(* Logix 5000 AddOnInstructionDefinition export EH_Dosimass_IOL; software revision 38.00 *)

TYPE EH_CommAOI_Data :
STRUCT
   Device_Comm_Error : BOOL;
   CommSuccess : BOOL;
   CommFailed : BOOL;
   CommTimeOut : BOOL;
   StateDone : BOOL;
   NewState : BOOL;
   OldState : SINT;
   PortSize : SINT;
   DevicePort : SINT;
   MaxState : SINT;
   State : SINT;
   VendorID : INT;
   DeviceID : DINT;
   CyclicData : INT[16];
   AcyclicData : DINT[8];
   ReplayIndex : INT;
   AOI_Diagnostic : DINT;
   ConnectionStatus : DINT;
   OutputData : INT[16];
END_STRUCT
END_TYPE

ADD_ON_INSTRUCTION EH_Dosimass_IOL   (* revision 1.1, vendor Endress+Hauser *)
// Dosimass D8AB Rev 1 IO-Link
// Revision note:
// 1.1 Changed the Datatype from Unsigned to Signed
// ZeroPoint adjustment update
// Add Disconnect check
// Add condition PulseSimulation
VAR_IN_OUT
   DataToSend : INT[10]; {required}
   CommAOIBusy : DINT; {required}
   ActiveComPort : DINT; {required}
   DeviceAOISendRequest : DINT; {required}
   CommError : INT; {required}
   DeviceData : EH_CommAOI_Data; {required}
END_VAR
VAR_INPUT
   iSetPulseSimulation : BOOL; {visible}
   iSimulationOnOff : BOOL; {visible}
   iAmountPulses : INT; {visible}
   iSetTotalizerPresetValue : BOOL; {visible}
   iTotalizer1PresetValue : REAL; {visible}
   iTotalizer_Hold : BOOL; {visible}
   iTotalizer_ResetTotalize : BOOL; {visible}
   iTotalizer_ResetHold : BOOL; {visible}
   iTotalizer_Totalize : BOOL; {visible}
   iParameterize : BOOL; {visible}
   iFlowDamping : REAL; {visible}
   iPressureShockSupression : REAL; {visible}
   iLowFlowCutoffValue : REAL; {visible}
   iFlowOverride : BOOL; {visible}
   iStartZeroPointAdjustment : BOOL; {visible}
END_VAR
VAR_OUTPUT
   qVendor_ID : DINT; {access Read Only, visible}
   qDevice_ID : DINT; {access Read Only, visible}
   qMassFlow : REAL; {visible}
   qDensity : REAL; {visible}
   qTemperature : REAL; {visible}
   qTotalizer1 : REAL; {access Read Only, visible}
   qExtendedDeviceStatus : INT; {access Read Only, visible}
   qZeroPointStatus : SINT; {access Read Only, visible}
   qReadProgress : SINT; {access Read Only, visible}
   qSSC1_1 : BOOL; {access Read Only, visible}
   qSSC1_2 : BOOL; {access Read Only, visible}
   qSSC2_1 : BOOL; {access Read Only, visible}
   qSSC2_2 : BOOL; {access Read Only, visible}
   qSSC3_1 : BOOL; {access Read Only, visible}
   qSSC3_2 : BOOL; {access Read Only, visible}
   qSSC4_1 : BOOL; {access Read Only, visible}
   qSSC4_2 : BOOL; {access Read Only, visible}
   qAOI_Diagnostic : DINT; {access Read Only, visible}
END_VAR
VAR_IN_OUT
   qAOI_Diagnostic_String : STRING; {required}
END_VAR
VAR_OUTPUT
   qActual_Diagnostics_Code : DINT; {access Read Only, visible}
END_VAR
VAR_IN_OUT
   qActual_Diagnostics_String : STRING; {required}
END_VAR
VAR_OUTPUT
   qLast_Diagnostics_Code : DINT; {visible}
END_VAR
VAR_IN_OUT
   qLast_Diagnostics_String : STRING; {required}
END_VAR
VAR_OUTPUT
   qCommError : DINT; {access None}
   qCommunicationBusy : DINT; {access Read Only, visible}
   qDeviceConnectionError : BOOL; {access Read Only, visible}
END_VAR
VAR
   Temp_DINT : DINT; {access None}
   CMD_Index : INT; {access None}
   CMD_Subindex : INT; {access None}
   CMD_ByteLength : INT; {access None}
   oldCondStatus : INT; {access None}
   SetSimulation : SINT; {access None}
   SetTotalizer : SINT; {access None}
   oldSetTotalizer : SINT; {access None}
   oldStartZeroPointAdjustment : SINT; {access None}
   Trigger : BOOL; {access None}
   CMD_Rd : BOOL; {access None}
   CMD_Wr : BOOL; {access None}
   SimulationDINT : DINT; {access None}
   AOI_Prio : BOOL; {access None}
   StateMin : DINT; {access None}
   firstTimeDone : BOOL; {access None}
   CondStatusChanged : BOOL; {access None}
   Calc_MassFlow : DINT; {access None}
   Calc_Density : DINT; {access None}
   Calc_Temperature : DINT; {access None}
   Calc_Totalizer1 : DINT; {access None}
   Calc_ExtendedDeviceStatus : DINT; {access None}
   CondStatusActive : BOOL; {access None}
   ActiveAOI : BOOL; {access None}
   TotActive : BOOL; {access None}
   Skip : BOOL; {access None}
   StartZeroPointAdjustment : SINT; {access None}
   Parameterize : SINT; {access None}
   oldParameterize : SINT; {access None}
   oldSetPulseSimulation : SINT; {access None}
   TotChanged : BOOL; {access None}
   DeviceID : DINT; {access None}
   SetPulseSimulation : SINT; {access None}
   zeroPointStatus : SINT; {access None}
   StartZeroPointAdjustmentChanged : BOOL; {access None}
   ParameterizeChanged : BOOL; {access None}
   PulseSimChanged : BOOL; {access None}
   TRUE : BOOL := 1; {access None}
   FALSE : BOOL; {access None}
   ParameterizeActive : BOOL; {access None}
   PulseSimActive : BOOL; {access None}
   ZeroPointActive : BOOL; {access None}
   StandardTimer : FBD_TIMER; {access None}
   temp_string1 : STRING; {access None}
   temp_string2 : STRING; {access None}
   onlyonce : BOOL; {access None}
END_VAR

ROUTINE Logic   (* structured text *)
// Picomag Communication via AL1323
   // =======================================================================
   // Endress+Hauser Digital Solutions
   // ©Copyright (2024) All Rights Reserved
   // =======================================================================
   // Name:                EH_Dosimass_IOL
   // Version:             1.1
   // Datum:               02.2026
   // Library:             01.01.00
   // Engineering:         Studio5000 V38.00.00
   // Author:              EH
   // =======================================================================
   
   qAOI_Diagnostic := DeviceData.AOI_Diagnostic;
   qCommunicationBusy := CommAOIBusy;
   DeviceID := 9729025;
   StateMin := 0;
   DeviceData.MaxState := 98;
   
   if DeviceData.DevicePort = 0 or DeviceData.DeviceID <> DeviceID or DeviceData.ConnectionStatus <> 1 then
   
   	qVendor_ID := DeviceData.VendorID;
   	qDevice_ID := DeviceData.DeviceID;
   	qMassFlow := 0;
   	qDensity := 0;
   	qTemperature := 0;
   	qTotalizer1	:= 0;
   	qExtendedDeviceStatus := 0;
   	qSSC1_1	:= FALSE;
   	qSSC1_2	:= FALSE;
   	qSSC2_1	:= FALSE;
   	qSSC2_2	:= FALSE;
   	qSSC3_1	:= FALSE;
   	qSSC3_2	:= FALSE;
   	qSSC4_1	:= FALSE;
   	qSSC4_2	:= FALSE;
   	qActual_Diagnostics_Code := 0;
   	qActual_Diagnostics_String := '';
   	qLast_Diagnostics_Code := 0;
   	qLast_Diagnostics_String := '';
   	qReadProgress := 0;
   	qZeroPointStatus := 0;
   	oldCondStatus := 0;
   	CondStatusChanged := FALSE;
   
   	if DeviceData.DevicePort = 0 then
   
   		qAOI_Diagnostic_String	:= 'Device Port is Zero';
   		DeviceData.AOI_Diagnostic.1 := TRUE;
   
   	elsif DeviceData.ConnectionStatus <> 1 then
   
   		qAOI_Diagnostic_String	:= 'No Device connected';
   		qDeviceConnectionError := TRUE;
   
   	elsif DeviceData.DeviceID <> DeviceID then
   
   		qAOI_Diagnostic_String	:= 'Wrong DeviceID';
   		DeviceData.AOI_Diagnostic.2 := TRUE;
   	end_if;
   
   else
   
   	if qActual_Diagnostics_Code = 0  then
   
   		qActual_Diagnostics_String	:= '--------';
   
   	end_if;
   
   	if qLast_Diagnostics_Code = 0 then
   
   		qLast_Diagnostics_String	:= '--------';
   
   	end_if;
   
   	qAOI_Diagnostic_String := '';
   	DeviceData.AOI_Diagnostic.1 := FALSE;
   	qDeviceConnectionError := FALSE;
   	DeviceData.AOI_Diagnostic.2  := FALSE;
   
   end_if;
   
   // Case device disconnected during communication to avoid blocking the communication
   if (DeviceData.AOI_Diagnostic.0 or qDeviceConnectionError or DeviceData.AOI_Diagnostic.2) and ActiveAOI and ActiveComPort = DeviceData.DevicePort and CommAOIBusy = 1 then
   
   	DeviceData.State := 0;
   	CommAOIBusy := 0;
   	DeviceAOISendRequest.[DeviceData.DevicePort] := 0;
   	ActiveComPort := 0;
   	ActiveAOI := 0;
   	DataToSend[0] := 0;
   	DataToSend[1] := 0;
   	DataToSend[2] := 0;
   	DataToSend[3] := 0;
   	DataToSend[4] := 0;
   	DataToSend[5] := 0;
   	DataToSend[6] := 0;
   	DataToSend[7] := 0;
   	DataToSend[8] := 0;
   	DataToSend[9] := 0;
   	DeviceData.StateDone := FALSE;
   	DeviceData.NewState := FALSE;
   	DeviceData.OldState := 0;
   	ActiveAOI := FALSE;
   
   end_if;
   
   if not DeviceData.AOI_Diagnostic.0
   	and not qDeviceConnectionError
   	and not DeviceData.AOI_Diagnostic.2
   	and DeviceData.DevicePort > 0 then
   
   	//*********************************
   	//Vendor ID
   	//*********************************
   
   		qVendor_ID := DeviceData.VendorID;
   
   	//*********************************
   	//Device ID
   	//*********************************
   
   		qDevice_ID := DeviceData.DeviceID;
   
   	//*********************************
   	// Dosimass
   	//*********************************
   
   		Calc_MassFlow				:= 0;
   		Calc_Density				:= 2;
   		Calc_Temperature			:= 4;
   		Calc_Totalizer1				:= 6;
   		Calc_ExtendedDeviceStatus	:= 8;
   
   	//*********************************
   	//Process MassFlow
   	//*********************************
   
   		Temp_DINT	 := DeviceData.CyclicData[Calc_MassFlow+1];
   		Temp_DINT.8	 := DeviceData.CyclicData[Calc_MassFlow+1].8;
   		Temp_DINT.9  := DeviceData.CyclicData[Calc_MassFlow+1].9;
   		Temp_DINT.10 := DeviceData.CyclicData[Calc_MassFlow+1].10;
   		Temp_DINT.11 := DeviceData.CyclicData[Calc_MassFlow+1].11;
   		Temp_DINT.12 := DeviceData.CyclicData[Calc_MassFlow+1].12;
   		Temp_DINT.13 := DeviceData.CyclicData[Calc_MassFlow+1].13;
   		Temp_DINT.14 := DeviceData.CyclicData[Calc_MassFlow+1].14;
   		Temp_DINT.15 := DeviceData.CyclicData[Calc_MassFlow+1].15;
   		Temp_DINT.16 := DeviceData.CyclicData[Calc_MassFlow].0;
   		Temp_DINT.17 := DeviceData.CyclicData[Calc_MassFlow].1;
   		Temp_DINT.18 := DeviceData.CyclicData[Calc_MassFlow].2;
   		Temp_DINT.19 := DeviceData.CyclicData[Calc_MassFlow].3;
   		Temp_DINT.20 := DeviceData.CyclicData[Calc_MassFlow].4;
   		Temp_DINT.21 := DeviceData.CyclicData[Calc_MassFlow].5;
   		Temp_DINT.22 := DeviceData.CyclicData[Calc_MassFlow].6;
   		Temp_DINT.23 := DeviceData.CyclicData[Calc_MassFlow].7;
   		Temp_DINT.24 := DeviceData.CyclicData[Calc_MassFlow].8;
   		Temp_DINT.25 := DeviceData.CyclicData[Calc_MassFlow].9;
   		Temp_DINT.26 := DeviceData.CyclicData[Calc_MassFlow].10;
   		Temp_DINT.27 := DeviceData.CyclicData[Calc_MassFlow].11;
   		Temp_DINT.28 := DeviceData.CyclicData[Calc_MassFlow].12;
   		Temp_DINT.29 := DeviceData.CyclicData[Calc_MassFlow].13;
   		Temp_DINT.30 := DeviceData.CyclicData[Calc_MassFlow].14;
   		Temp_DINT.31 := DeviceData.CyclicData[Calc_MassFlow].15;
   
   		COP(Temp_DINT,qMassFlow,1);
   
   	//*********************************
   	//Process Data Density
   	//*********************************
   
   		Temp_DINT	 := DeviceData.CyclicData[Calc_Density+1];
   		Temp_DINT.8	 := DeviceData.CyclicData[Calc_Density+1].8;
   		Temp_DINT.9	 := DeviceData.CyclicData[Calc_Density+1].9;
   		Temp_DINT.10 := DeviceData.CyclicData[Calc_Density+1].10;
   		Temp_DINT.11 := DeviceData.CyclicData[Calc_Density+1].11;
   		Temp_DINT.12 := DeviceData.CyclicData[Calc_Density+1].12;
   		Temp_DINT.13 := DeviceData.CyclicData[Calc_Density+1].13;
   		Temp_DINT.14 := DeviceData.CyclicData[Calc_Density+1].14;
   		Temp_DINT.15 := DeviceData.CyclicData[Calc_Density+1].15;
   		Temp_DINT.16 := DeviceData.CyclicData[Calc_Density].0;
   		Temp_DINT.17 := DeviceData.CyclicData[Calc_Density].1;
   		Temp_DINT.18 := DeviceData.CyclicData[Calc_Density].2;
   		Temp_DINT.19 := DeviceData.CyclicData[Calc_Density].3;
   		Temp_DINT.20 := DeviceData.CyclicData[Calc_Density].4;
   		Temp_DINT.21 := DeviceData.CyclicData[Calc_Density].5;
   		Temp_DINT.22 := DeviceData.CyclicData[Calc_Density].6;
   		Temp_DINT.23 := DeviceData.CyclicData[Calc_Density].7;
   		Temp_DINT.24 := DeviceData.CyclicData[Calc_Density].8;
   		Temp_DINT.25 := DeviceData.CyclicData[Calc_Density].9;
   		Temp_DINT.26 := DeviceData.CyclicData[Calc_Density].10;
   		Temp_DINT.27 := DeviceData.CyclicData[Calc_Density].11;
   		Temp_DINT.28 := DeviceData.CyclicData[Calc_Density].12;
   		Temp_DINT.29 := DeviceData.CyclicData[Calc_Density].13;
   		Temp_DINT.30 := DeviceData.CyclicData[Calc_Density].14;
   		Temp_DINT.31 := DeviceData.CyclicData[Calc_Density].15;
   
   		COP(Temp_DINT,qDensity,1);
   
   	//*********************************
   	//Process Data Temperature
   	//*********************************
   
   		Temp_DINT	 := DeviceData.CyclicData[Calc_Temperature+1];
   		Temp_DINT.8	 := DeviceData.CyclicData[Calc_Temperature+1].8;
   		Temp_DINT.9	 := DeviceData.CyclicData[Calc_Temperature+1].9;
   		Temp_DINT.10 := DeviceData.CyclicData[Calc_Temperature+1].10;
   		Temp_DINT.11 := DeviceData.CyclicData[Calc_Temperature+1].11;
   		Temp_DINT.12 := DeviceData.CyclicData[Calc_Temperature+1].12;
   		Temp_DINT.13 := DeviceData.CyclicData[Calc_Temperature+1].13;
   		Temp_DINT.14 := DeviceData.CyclicData[Calc_Temperature+1].14;
   		Temp_DINT.15 := DeviceData.CyclicData[Calc_Temperature+1].15;
   		Temp_DINT.16 := DeviceData.CyclicData[Calc_Temperature].0;
   		Temp_DINT.17 := DeviceData.CyclicData[Calc_Temperature].1;
   		Temp_DINT.18 := DeviceData.CyclicData[Calc_Temperature].2;
   		Temp_DINT.19 := DeviceData.CyclicData[Calc_Temperature].3;
   		Temp_DINT.20 := DeviceData.CyclicData[Calc_Temperature].4;
   		Temp_DINT.21 := DeviceData.CyclicData[Calc_Temperature].5;
   		Temp_DINT.22 := DeviceData.CyclicData[Calc_Temperature].6;
   		Temp_DINT.23 := DeviceData.CyclicData[Calc_Temperature].7;
   		Temp_DINT.24 := DeviceData.CyclicData[Calc_Temperature].8;
   		Temp_DINT.25 := DeviceData.CyclicData[Calc_Temperature].9;
   		Temp_DINT.26 := DeviceData.CyclicData[Calc_Temperature].10;
   		Temp_DINT.27 := DeviceData.CyclicData[Calc_Temperature].11;
   		Temp_DINT.28 := DeviceData.CyclicData[Calc_Temperature].12;
   		Temp_DINT.29 := DeviceData.CyclicData[Calc_Temperature].13;
   		Temp_DINT.30 := DeviceData.CyclicData[Calc_Temperature].14;
   		Temp_DINT.31 := DeviceData.CyclicData[Calc_Temperature].15;
   
   		COP(Temp_DINT,qTemperature,1);
   
   	//*********************************
   	// Process Parameter Totalizer1
   	//*********************************
   
   		Temp_DINT	 := DeviceData.CyclicData[Calc_Totalizer1+1];
   		Temp_DINT.8  := DeviceData.CyclicData[Calc_Totalizer1+1].8;
   		Temp_DINT.9  := DeviceData.CyclicData[Calc_Totalizer1+1].9;
   		Temp_DINT.10 := DeviceData.CyclicData[Calc_Totalizer1+1].10;
   		Temp_DINT.11 := DeviceData.CyclicData[Calc_Totalizer1+1].11;
   		Temp_DINT.12 := DeviceData.CyclicData[Calc_Totalizer1+1].12;
   		Temp_DINT.13 := DeviceData.CyclicData[Calc_Totalizer1+1].13;
   		Temp_DINT.14 := DeviceData.CyclicData[Calc_Totalizer1+1].14;
   		Temp_DINT.15 := DeviceData.CyclicData[Calc_Totalizer1+1].15;
   		Temp_DINT.16 := DeviceData.CyclicData[Calc_Totalizer1].0;
   		Temp_DINT.17 := DeviceData.CyclicData[Calc_Totalizer1].1;
   		Temp_DINT.18 := DeviceData.CyclicData[Calc_Totalizer1].2;
   		Temp_DINT.19 := DeviceData.CyclicData[Calc_Totalizer1].3;
   		Temp_DINT.20 := DeviceData.CyclicData[Calc_Totalizer1].4;
   		Temp_DINT.21 := DeviceData.CyclicData[Calc_Totalizer1].5;
   		Temp_DINT.22 := DeviceData.CyclicData[Calc_Totalizer1].6;
   		Temp_DINT.23 := DeviceData.CyclicData[Calc_Totalizer1].7;
   		Temp_DINT.24 := DeviceData.CyclicData[Calc_Totalizer1].8;
   		Temp_DINT.25 := DeviceData.CyclicData[Calc_Totalizer1].9;
   		Temp_DINT.26 := DeviceData.CyclicData[Calc_Totalizer1].10;
   		Temp_DINT.27 := DeviceData.CyclicData[Calc_Totalizer1].11;
   		Temp_DINT.28 := DeviceData.CyclicData[Calc_Totalizer1].12;
   		Temp_DINT.29 := DeviceData.CyclicData[Calc_Totalizer1].13;
   		Temp_DINT.30 := DeviceData.CyclicData[Calc_Totalizer1].14;
   		Temp_DINT.31 := DeviceData.CyclicData[Calc_Totalizer1].15;
   
   		COP(Temp_DINT,qTotalizer1,1);
   
   	//*********************************
   	// Extended device Status
   	//*********************************
   
   		qExtendedDeviceStatus.0 := DeviceData.CyclicData[Calc_ExtendedDeviceStatus].8;
   		qExtendedDeviceStatus.1 := DeviceData.CyclicData[Calc_ExtendedDeviceStatus].9;
   		qExtendedDeviceStatus.2 := DeviceData.CyclicData[Calc_ExtendedDeviceStatus].10;
   		qExtendedDeviceStatus.3 := DeviceData.CyclicData[Calc_ExtendedDeviceStatus].11;
   		qExtendedDeviceStatus.4 := DeviceData.CyclicData[Calc_ExtendedDeviceStatus].12;
   		qExtendedDeviceStatus.5 := DeviceData.CyclicData[Calc_ExtendedDeviceStatus].13;
   		qExtendedDeviceStatus.6 := DeviceData.CyclicData[Calc_ExtendedDeviceStatus].14;
   		qExtendedDeviceStatus.7 := DeviceData.CyclicData[Calc_ExtendedDeviceStatus].15;
   
   	//*********************************
   	// Process Parameter SSC
   	//*********************************
   
   		qSSC1_1 := DeviceData.CyclicData[Calc_ExtendedDeviceStatus].0;
   		qSSC1_2 := DeviceData.CyclicData[Calc_ExtendedDeviceStatus].1;
   
   		qSSC2_1 := DeviceData.CyclicData[Calc_ExtendedDeviceStatus].2;
   		qSSC2_2 := DeviceData.CyclicData[Calc_ExtendedDeviceStatus].3;
   
   		qSSC3_1 := DeviceData.CyclicData[Calc_ExtendedDeviceStatus].4;
   		qSSC3_2 := DeviceData.CyclicData[Calc_ExtendedDeviceStatus].5;
   
   		qSSC4_1 := DeviceData.CyclicData[Calc_ExtendedDeviceStatus].6;
   		qSSC4_2 := DeviceData.CyclicData[Calc_ExtendedDeviceStatus].7;
   
   	//*********************************
   	// Process Output Parameter
   	//*********************************
   
   		DeviceData.OutputData[0].5 := iFlowOverride;
   		DeviceData.OutputData[0].6 := iTotalizer_Hold;
   		DeviceData.OutputData[0].7 := iTotalizer_ResetTotalize;
   		DeviceData.OutputData[0].8 := iTotalizer_ResetHold;
   		DeviceData.OutputData[0].9 := iTotalizer_Totalize;
   
   	//*********************************
   	// Checking for Changed Status
   	//*********************************
   
   		SetTotalizer.0 := iSetTotalizerPresetValue;
   		Parameterize.0 := iParameterize;
   		StartZeroPointAdjustment.0 := iStartZeroPointAdjustment;
   		SetPulseSimulation.0 := iSetPulseSimulation;
   
   		if oldCondStatus <> qExtendedDeviceStatus and not CondStatusChanged then
   
   			CondStatusChanged := TRUE;
   			oldCondStatus := qExtendedDeviceStatus;
   
   		end_if;
   
   		if oldSetPulseSimulation <> SetPulseSimulation and not PulseSimChanged then
   
   			if oldSetPulseSimulation < SetPulseSimulation then
   
   				PulseSimChanged := TRUE;
   
   			end_if;
   
   			oldSetPulseSimulation := SetPulseSimulation;
   
   		end_if;
   
   		if oldStartZeroPointAdjustment <> StartZeroPointAdjustment and not StartZeroPointAdjustmentChanged then
   
   			if oldStartZeroPointAdjustment < StartZeroPointAdjustment then
   
   				StartZeroPointAdjustmentChanged := TRUE;
   
   			end_if;
   
   			oldStartZeroPointAdjustment := StartZeroPointAdjustment;
   
   		end_if;
   
   		if oldParameterize <> Parameterize and not ParameterizeChanged then
   
   			if oldParameterize < Parameterize then
   
   				ParameterizeChanged := TRUE;
   
   			end_if;
   
   			oldParameterize := Parameterize;
   
   		end_if;
   
   		if oldSetTotalizer <> SetTotalizer and not TotChanged then
   
   			if oldSetTotalizer < SetTotalizer then
   
   				TotChanged := TRUE;
   
   			end_if;
   
   			oldSetTotalizer := SetTotalizer;
   
   		end_if;
   
   		if CondStatusChanged
   		and not ActiveAOI
   		and not CondStatusActive
   		and not Skip then
   
   			DeviceAOISendRequest.[DeviceData.DevicePort] := TRUE;
   			CondStatusActive := TRUE;
   			Skip := TRUE;
   
   		elsif PulseSimChanged
   			and not ActiveAOI
   			and not PulseSimActive
   			and not Skip then
   
   			DeviceAOISendRequest.[DeviceData.DevicePort] := TRUE;
   			PulseSimActive := TRUE;
   			Skip := TRUE;
   
   		elsif TotChanged
   			and not ActiveAOI
   			and not TotActive
   			and not Skip then
   
   			DeviceAOISendRequest.[DeviceData.DevicePort] := TRUE;
   			TotActive := TRUE;
   			Skip := TRUE;
   
   		elsif StartZeroPointAdjustmentChanged
   			and not ActiveAOI
   			and not ZeroPointActive
   			and not Skip then
   
   			DeviceAOISendRequest.[DeviceData.DevicePort] := TRUE;
   			ZeroPointActive := TRUE;
   			Skip := TRUE;
   
   		elsif ParameterizeChanged
   			and not ActiveAOI
   			and not ParameterizeActive
   			and not Skip then
   
   			DeviceAOISendRequest.[DeviceData.DevicePort] := TRUE;
   			ParameterizeActive := TRUE;
   			Skip := TRUE;
   
   		end_if;
   
   		if ActiveComPort = DeviceData.DevicePort then
   
   			AOI_Prio :=TRUE;
   
   		else
   
   			AOI_Prio := FALSE;
   
   		end_if;
   
   		if (PulseSimActive or TotActive or CondStatusActive or ParameterizeActive or ZeroPointActive) and CommAOIBusy = 1  and DeviceData.State = 0 and AOI_Prio and not ActiveAOI then
   
   			ActiveAOI := TRUE;
   			Skip := FALSE;
   
   		end_if;
   
   		qCommunicationBusy := CommAOIBusy;
   		qAOI_Diagnostic :=DeviceData.AOI_Diagnostic;
   
   	//*********************************
   	// States for Execution
   	//*********************************
   
   	if ActiveAOI or DeviceData.State = DeviceData.MaxState then
   
   	case DeviceData.State of
   
   		//*********************************
   		0: // Idle
   		//*********************************
   
   			// Initializing
   			Trigger := FALSE;
   			CMD_Index := 0;
   			CMD_Subindex := 0;
   			CMD_Wr := FALSE;
   			CMD_Rd := FALSE;
   		    CMD_ByteLength := 0;
   
   			if DeviceData.DevicePort = ActiveComPort then
   					DeviceData.CommSuccess := FALSE;
   					DeviceData.CommTimeOut := FALSE;
   					DeviceData.NewState := TRUE;
   					DeviceData.StateDone := FALSE;
   			end_if;
   
   			// Wait for trigger
   			if ParameterizeActive then
   
   				DeviceData.AOI_Diagnostic := 0;
   				DeviceData.State := 6;
   
   			elsif PulseSimActive then
   
   				DeviceData.AOI_Diagnostic := 0;
   				DeviceData.State := 15;
   
   			elsif TotActive then
   				DeviceData.AOI_Diagnostic := 0;
   				DeviceData.State := 20;
   
   			elsif ZeroPointActive then
   
   				DeviceData.AOI_Diagnostic := 0;
   				qReadProgress := 0;
   				qZeroPointStatus := 0;
   				DeviceData.State := 30;
   
   			elsif CondStatusChanged then
   
   				DeviceData.State := 90;
   
   			end_if;
   
   		//*********************************
   		6: // Set Flow Damping
   		//*********************************
   
   			CMD_Index := 2129;
   			CMD_Subindex := 0;
   			CMD_Wr := TRUE;
   			CMD_Rd := FALSE;
   			CMD_ByteLength := 4;
   			DataToSend[6]:= 0;
   			DataToSend[7]:= 0;
   
   			COP(iFlowDamping,SimulationDINT,1);		// Copy the Bits from the Real in a DINT
   
   			DataToSend[6].0 :=  SimulationDINT.24;
   			DataToSend[6].1 :=  SimulationDINT.25;
   			DataToSend[6].2 :=  SimulationDINT.26;
   			DataToSend[6].3 :=  SimulationDINT.27;
   			DataToSend[6].4 :=  SimulationDINT.28;
   			DataToSend[6].5 :=  SimulationDINT.29;
   			DataToSend[6].6 :=  SimulationDINT.30;
   			DataToSend[6].7 :=  SimulationDINT.31;
   			DataToSend[6].8 :=  SimulationDINT.16;
   			DataToSend[6].9 :=  SimulationDINT.17;
   			DataToSend[6].10 := SimulationDINT.18;
   			DataToSend[6].11 := SimulationDINT.19;
   			DataToSend[6].12 := SimulationDINT.20;
   			DataToSend[6].13 := SimulationDINT.21;
   			DataToSend[6].14 := SimulationDINT.22;
   			DataToSend[6].15 := SimulationDINT.23;
   			DataToSend[7].0  := SimulationDINT.8;
   			DataToSend[7].1  := SimulationDINT.9;
   			DataToSend[7].2  := SimulationDINT.10;
   			DataToSend[7].3  := SimulationDINT.11;
   			DataToSend[7].4  := SimulationDINT.12;
   			DataToSend[7].5  := SimulationDINT.13;
   			DataToSend[7].6  := SimulationDINT.14;
   			DataToSend[7].7  := SimulationDINT.15;
   			DataToSend[7].8  := SimulationDINT.0;
   			DataToSend[7].9  := SimulationDINT.1;
   			DataToSend[7].10 := SimulationDINT.2;
   			DataToSend[7].11 := SimulationDINT.3;
   			DataToSend[7].12 := SimulationDINT.4;
   			DataToSend[7].13 := SimulationDINT.5;
   			DataToSend[7].14 := SimulationDINT.6;
   			DataToSend[7].15 := SimulationDINT.7;
   
   			Trigger := TRUE;
   
   			if DeviceData.NewState then
   
   				DeviceData.StateDone := TRUE;
   
   			end_if;
   
   			if DeviceData.CommSuccess and DeviceData.ReplayIndex = CMD_Index then
   
   				Trigger := FALSE;
   				DeviceData.OldState := DeviceData.State;
   				DeviceData.State := DeviceData.State + 1;
   				DeviceData.CommSuccess := FALSE;
   				DeviceData.AcyclicData[0] := 0;
   				DeviceData.NewState := TRUE;
   
   			elsif DeviceData.CommTimeOut then
   
   				temp_string1 := 'Error in step ';
   				Temp_DINT := DeviceData.State;
   				DTOS(Temp_DINT, temp_string2);
   				CONCAT(temp_string1, temp_string2, qAOI_Diagnostic_String);
   
   				DeviceData.OldState := DeviceData.State;
   				DeviceData.State := DeviceData.MaxState;	//Check State
   				DeviceData.CommTimeOut := FALSE;
   				DeviceData.AcyclicData[0] := 0;
   				DeviceData.NewState := TRUE;
   
   			end_if;
   
   		//*********************************
   		7: // Set pressure shock supression
   		//*********************************
   
   			CMD_Index := 2108;
   			CMD_Subindex := 0;
   			CMD_Wr := TRUE;
   			CMD_Rd := FALSE;
   			CMD_ByteLength := 4;
   			DataToSend[6]:= 0;
   			DataToSend[7]:= 0;
   
   			COP(iPressureShockSupression,SimulationDINT,1);		// Copy the Bits from the Real in a DINT
   
   			DataToSend[6].0 :=  SimulationDINT.24;
   			DataToSend[6].1 :=  SimulationDINT.25;
   			DataToSend[6].2 :=  SimulationDINT.26;
   			DataToSend[6].3 :=  SimulationDINT.27;
   			DataToSend[6].4 :=  SimulationDINT.28;
   			DataToSend[6].5 :=  SimulationDINT.29;
   			DataToSend[6].6 :=  SimulationDINT.30;
   			DataToSend[6].7 :=  SimulationDINT.31;
   			DataToSend[6].8 :=  SimulationDINT.16;
   			DataToSend[6].9 :=  SimulationDINT.17;
   			DataToSend[6].10 := SimulationDINT.18;
   			DataToSend[6].11 := SimulationDINT.19;
   			DataToSend[6].12 := SimulationDINT.20;
   			DataToSend[6].13 := SimulationDINT.21;
   			DataToSend[6].14 := SimulationDINT.22;
   			DataToSend[6].15 := SimulationDINT.23;
   			DataToSend[7].0  := SimulationDINT.8;
   			DataToSend[7].1  := SimulationDINT.9;
   			DataToSend[7].2  := SimulationDINT.10;
   			DataToSend[7].3  := SimulationDINT.11;
   			DataToSend[7].4  := SimulationDINT.12;
   			DataToSend[7].5  := SimulationDINT.13;
   			DataToSend[7].6  := SimulationDINT.14;
   			DataToSend[7].7  := SimulationDINT.15;
   			DataToSend[7].8  := SimulationDINT.0;
   			DataToSend[7].9  := SimulationDINT.1;
   			DataToSend[7].10 := SimulationDINT.2;
   			DataToSend[7].11 := SimulationDINT.3;
   			DataToSend[7].12 := SimulationDINT.4;
   			DataToSend[7].13 := SimulationDINT.5;
   			DataToSend[7].14 := SimulationDINT.6;
   			DataToSend[7].15 := SimulationDINT.7;
   
   			Trigger := TRUE;
   
   			if DeviceData.NewState then
   
   				DeviceData.StateDone := TRUE;
   
   			end_if;
   
   			if DeviceData.CommSuccess and DeviceData.ReplayIndex = CMD_Index then
   
   				Trigger := FALSE;
   				DeviceData.OldState := DeviceData.State;
   				DeviceData.State := 10;
   				DeviceData.CommSuccess := FALSE;
   				DeviceData.AcyclicData[0] := 0;
   				DeviceData.NewState := TRUE;
   
   			elsif DeviceData.CommTimeOut then
   
   				temp_string1 := 'Error in step ';
   				Temp_DINT := DeviceData.State;
   				DTOS(Temp_DINT, temp_string2);
   				CONCAT(temp_string1, temp_string2, qAOI_Diagnostic_String);
   
   				DeviceData.OldState := DeviceData.State;
   				DeviceData.State := DeviceData.MaxState;	//Check State
   				DeviceData.CommTimeOut := FALSE;
   				DeviceData.AcyclicData[0] := 0;
   				DeviceData.NewState := TRUE;
   
   			end_if;
   
   		//*********************************
   		10: // Low flow cut off value
   		//*********************************
   
   			CMD_Index := 2067;
   			CMD_Subindex := 0;
   			CMD_Wr := TRUE;
   			CMD_Rd := FALSE;
   			CMD_ByteLength := 4;
   			DataToSend[6]:= 0;
   			DataToSend[7]:= 0;
   
   
   			COP(iLowFlowCutoffValue ,SimulationDINT,1);		// Copy the Bits from the Real in a DINT
   
   			DataToSend[6].0 :=  SimulationDINT.24;
   			DataToSend[6].1 :=  SimulationDINT.25;
   			DataToSend[6].2 :=  SimulationDINT.26;
   			DataToSend[6].3 :=  SimulationDINT.27;
   			DataToSend[6].4 :=  SimulationDINT.28;
   			DataToSend[6].5 :=  SimulationDINT.29;
   			DataToSend[6].6 :=  SimulationDINT.30;
   			DataToSend[6].7 :=  SimulationDINT.31;
   			DataToSend[6].8 :=  SimulationDINT.16;
   			DataToSend[6].9 :=  SimulationDINT.17;
   			DataToSend[6].10 := SimulationDINT.18;
   			DataToSend[6].11 := SimulationDINT.19;
   			DataToSend[6].12 := SimulationDINT.20;
   			DataToSend[6].13 := SimulationDINT.21;
   			DataToSend[6].14 := SimulationDINT.22;
   			DataToSend[6].15 := SimulationDINT.23;
   			DataToSend[7].0  := SimulationDINT.8;
   			DataToSend[7].1  := SimulationDINT.9;
   			DataToSend[7].2  := SimulationDINT.10;
   			DataToSend[7].3  := SimulationDINT.11;
   			DataToSend[7].4  := SimulationDINT.12;
   			DataToSend[7].5  := SimulationDINT.13;
   			DataToSend[7].6  := SimulationDINT.14;
   			DataToSend[7].7  := SimulationDINT.15;
   			DataToSend[7].8  := SimulationDINT.0;
   			DataToSend[7].9  := SimulationDINT.1;
   			DataToSend[7].10 := SimulationDINT.2;
   			DataToSend[7].11 := SimulationDINT.3;
   			DataToSend[7].12 := SimulationDINT.4;
   			DataToSend[7].13 := SimulationDINT.5;
   			DataToSend[7].14 := SimulationDINT.6;
   			DataToSend[7].15 := SimulationDINT.7;
   
   			Trigger := TRUE;
   
   			if DeviceData.NewState then
   
   				DeviceData.StateDone := TRUE;
   
   			end_if;
   
   			if DeviceData.CommSuccess and DeviceData.ReplayIndex = CMD_Index then
   
   				Trigger := FALSE;
   				DeviceData.OldState := DeviceData.State;
   				DeviceData.State := DeviceData.MaxState;
   				DeviceData.CommSuccess := FALSE;
   				DeviceData.AcyclicData[0] := 0;
   				DeviceData.NewState := TRUE;
   
   			elsif DeviceData.CommTimeOut then
   
   				temp_string1 := 'Error in step ';
   				Temp_DINT := DeviceData.State;
   				DTOS(Temp_DINT, temp_string2);
   				CONCAT(temp_string1, temp_string2, qAOI_Diagnostic_String);
   
   				DeviceData.OldState := DeviceData.State;
   				DeviceData.State := DeviceData.MaxState;	//Check State
   				DeviceData.CommTimeOut := FALSE;
   				DeviceData.AcyclicData[0] := 0;
   				DeviceData.NewState := TRUE;
   
   			end_if;
   
   		//***************************************
   		15: // Set pulse simulation to count down
   		//***************************************
   
   			CMD_Index := 372;
   			CMD_Subindex := 0;
   			CMD_Wr := TRUE;								// Only Read or Write can be active = 1
   			CMD_Rd := FALSE;
   			CMD_ByteLength := 2;
   
   			DataToSend[6] := 0;
   			DataToSend[7] := 0;
   
   			if iSimulationOnOff then
   
   				DataToSend[6].8 := TRUE;
   				DataToSend[7] := 0;
   
   			else
   
   				DataToSend[6] := 0;
   				DataToSend[7] := 0;
   
   			end_if;
   
   			Trigger := TRUE;
   
   			if DeviceData.NewState then
   
   				DeviceData.StateDone := TRUE;
   
   			end_if;
   
   			if  DeviceData.CommSuccess and DeviceData.ReplayIndex = CMD_Index then
   
   				Trigger := FALSE;
   				DeviceData.OldState := DeviceData.State;
   				if iSimulationOnOff then
   					DeviceData.State := DeviceData.State + 1;
   				else
   					DeviceData.State := DeviceData.MaxState;
   				end_if;
   				DeviceData.CommSuccess := FALSE;
   				DeviceData.AcyclicData[0] := 0;
   				DeviceData.NewState := TRUE;
   
   			elsif DeviceData.CommTimeOut then
   
   				temp_string1 := 'Error in step ';
   				Temp_DINT := DeviceData.State;
   				DTOS(Temp_DINT, temp_string2);
   				CONCAT(temp_string1, temp_string2, qAOI_Diagnostic_String);
   
   				DeviceData.OldState := DeviceData.State;
   				DeviceData.State := DeviceData.MaxState;
   				DeviceData.CommTimeOut := FALSE;
   				DeviceData.AcyclicData[0] := 0;
   				DeviceData.NewState := TRUE;
   
   			end_if;
   
   
   		//*********************************
   		16: // Set pulse simulation value
   		//*********************************
   
   			CMD_Index := 373;
   			CMD_Subindex := 0;
   			CMD_Wr := TRUE;
   			CMD_Rd := FALSE;
   			CMD_ByteLength := 2;
   			DataToSend[6]:= 0;
   			DataToSend[7]:= 0;
   
   		 	COP(iAmountPulses,SimulationDINT,1);		// Copy the Bits from the Real in a DINT
   
   			DataToSend[6].0 :=  SimulationDINT.8;
   			DataToSend[6].1 :=  SimulationDINT.9;
   			DataToSend[6].2 :=  SimulationDINT.10;
   			DataToSend[6].3 :=  SimulationDINT.11;
   			DataToSend[6].4 :=  SimulationDINT.12;
   			DataToSend[6].5 :=  SimulationDINT.13;
   			DataToSend[6].6 :=  SimulationDINT.14;
   			DataToSend[6].7 :=  SimulationDINT.15;
   			DataToSend[6].8 :=  SimulationDINT.0;
   			DataToSend[6].9 :=  SimulationDINT.1;
   			DataToSend[6].10 := SimulationDINT.2;
   			DataToSend[6].11 := SimulationDINT.3;
   			DataToSend[6].12 := SimulationDINT.4;
   			DataToSend[6].13 := SimulationDINT.5;
   			DataToSend[6].14 := SimulationDINT.6;
   			DataToSend[6].15 := SimulationDINT.7;
   
   			Trigger := TRUE;
   
   			if DeviceData.NewState then
   
   				DeviceData.StateDone := TRUE;
   
   			end_if;
   
   			if DeviceData.CommSuccess and DeviceData.ReplayIndex = CMD_Index then
   
   				Trigger := FALSE;
   				DeviceData.OldState := DeviceData.State;
   				DeviceData.State := DeviceData.MaxState;
   				DeviceData.CommSuccess := FALSE;
   				DeviceData.AcyclicData[0] := 0;
   				DeviceData.NewState := TRUE;
   
   			elsif DeviceData.CommTimeOut then
   
   				temp_string1 := 'Error in step ';
   				Temp_DINT := DeviceData.State;
   				DTOS(Temp_DINT, temp_string2);
   				CONCAT(temp_string1, temp_string2, qAOI_Diagnostic_String);
   
   				DeviceData.OldState := DeviceData.State;
   				DeviceData.State := DeviceData.MaxState;	//Check State
   				DeviceData.CommTimeOut := FALSE;
   				DeviceData.AcyclicData[0] := 0;
   				DeviceData.NewState := TRUE;
   
   			end_if;
   
   
   		//*********************************
   		20: // Totalizer 1 preset value
   		//*********************************
   
   			CMD_Index := 2103;
   			CMD_Subindex := 0;
   			CMD_Wr := TRUE;								// Only Read or Write can be active = 1
   			CMD_Rd := FALSE;
   			CMD_ByteLength := 4;
   			DataToSend[6]:= 0;
   			DataToSend[7]:= 0;
   
   		 	COP(iTotalizer1PresetValue,SimulationDINT,1); // Copy the Bits from the Real in a DINT
   
   			DataToSend[6].0 :=  SimulationDINT.24;
   			DataToSend[6].1 :=  SimulationDINT.25;
   			DataToSend[6].2 :=  SimulationDINT.26;
   			DataToSend[6].3 :=  SimulationDINT.27;
   			DataToSend[6].4 :=  SimulationDINT.28;
   			DataToSend[6].5 :=  SimulationDINT.29;
   			DataToSend[6].6 :=  SimulationDINT.30;
   			DataToSend[6].7 :=  SimulationDINT.31;
   			DataToSend[6].8 :=  SimulationDINT.16;
   			DataToSend[6].9 :=  SimulationDINT.17;
   			DataToSend[6].10 := SimulationDINT.18;
   			DataToSend[6].11 := SimulationDINT.19;
   			DataToSend[6].12 := SimulationDINT.20;
   			DataToSend[6].13 := SimulationDINT.21;
   			DataToSend[6].14 := SimulationDINT.22;
   			DataToSend[6].15 := SimulationDINT.23;
   			DataToSend[7].0  := SimulationDINT.8;
   			DataToSend[7].1  := SimulationDINT.9;
   			DataToSend[7].2  := SimulationDINT.10;
   			DataToSend[7].3  := SimulationDINT.11;
   			DataToSend[7].4  := SimulationDINT.12;
   			DataToSend[7].5  := SimulationDINT.13;
   			DataToSend[7].6  := SimulationDINT.14;
   			DataToSend[7].7  := SimulationDINT.15;
   			DataToSend[7].8  := SimulationDINT.0;
   			DataToSend[7].9  := SimulationDINT.1;
   			DataToSend[7].10 := SimulationDINT.2;
   			DataToSend[7].11 := SimulationDINT.3;
   			DataToSend[7].12 := SimulationDINT.4;
   			DataToSend[7].13 := SimulationDINT.5;
   			DataToSend[7].14 := SimulationDINT.6;
   			DataToSend[7].15 := SimulationDINT.7;
   
   			Trigger := TRUE;
   
   			if DeviceData.NewState then
   
   				DeviceData.StateDone := TRUE;
   
   			end_if;
   
   			if  DeviceData.CommSuccess and DeviceData.ReplayIndex = CMD_Index then
   
   				Trigger := FALSE;
   				DeviceData.OldState := DeviceData.State;
   				DeviceData.State := DeviceData.State + 1;
   				DeviceData.CommSuccess := FALSE;
   				DeviceData.AcyclicData[0] := 0;
   				DeviceData.NewState := TRUE;
   
   			 elsif DeviceData.CommTimeOut then
   
   				temp_string1 := 'Error in step ';
   				Temp_DINT := DeviceData.State;
   				DTOS(Temp_DINT, temp_string2);
   				CONCAT(temp_string1, temp_string2, qAOI_Diagnostic_String);
   
   				DeviceData.OldState := DeviceData.State;
   				DeviceData.State := DeviceData.MaxState;	//Check State
   				DeviceData.CommTimeOut := FALSE;
   				DeviceData.AcyclicData[0] := 0;
   				DeviceData.NewState := TRUE;
   
   			end_if;
   
   		//*********************************
   		21: // Totalizer 1 control
   		//*********************************
   
   			CMD_Index := 2100;
   			CMD_Subindex := 0;
   			CMD_Wr := TRUE;
   			CMD_Rd := FALSE;
   			CMD_ByteLength := 2;
   			DataToSend[6]:= 0;
   			DataToSend[7]:= 0;
   
   			DataToSend[6].9:= 1; // Preset + hold
   
   			Trigger := TRUE;
   
   			if DeviceData.NewState then
   
   				DeviceData.StateDone := TRUE;
   
   			end_if;
   
   			if  DeviceData.CommSuccess and DeviceData.ReplayIndex = CMD_Index then
   
   				Trigger := FALSE;
   				DeviceData.OldState := DeviceData.State;
   				DeviceData.State := DeviceData.MaxState;
   				DeviceData.CommSuccess := FALSE;
   				DeviceData.AcyclicData[0] := 0;
   				DeviceData.NewState := TRUE;
   
   			elsif DeviceData.CommTimeOut then
   
   				temp_string1 := 'Error in step ';
   				Temp_DINT := DeviceData.State;
   				DTOS(Temp_DINT, temp_string2);
   				CONCAT(temp_string1, temp_string2, qAOI_Diagnostic_String);
   
   				DeviceData.OldState := DeviceData.State;
   				DeviceData.State := DeviceData.MaxState;
   				DeviceData.CommTimeOut := FALSE;
   				DeviceData.AcyclicData[0] := 0;
   				DeviceData.NewState := TRUE;
   
   			end_if;
   
   		//***************************************
   	    30: // Read zero point adjustment status
   		//***************************************
   
   			CMD_Index := 2196;
   			CMD_Subindex := 0;
   			CMD_Wr := FALSE;
   			CMD_Rd := TRUE;
   			CMD_ByteLength := 2;
   			Trigger := TRUE;
   
   			if DeviceData.NewState then
   
   				DeviceData.StateDone := TRUE;
   
   			end_if;
   
   			if  DeviceData.CommSuccess and DeviceData.ReplayIndex = CMD_Index then
   
   				if DeviceData.AcyclicData[0] = 8 then
   
   					DeviceData.State := DeviceData.MaxState; // Zero Point already in progress
   					qAOI_Diagnostic_String := 'Zero point adjustement already in progress';
   
   				else
   
   					DeviceData.State := DeviceData.State + 1;
   
   				end_if;
   
   			Trigger := FALSE;
   			DeviceData.CommSuccess := FALSE;
   			DeviceData.AcyclicData[0] := 0;
   			DeviceData.NewState := TRUE;
   
   		elsif DeviceData.CommTimeOut then
   
   			temp_string1 := 'Error in step ';
   			Temp_DINT := DeviceData.State;
   			DTOS(Temp_DINT, temp_string2);
   			CONCAT(temp_string1, temp_string2, qAOI_Diagnostic_String);
   
   			DeviceData.OldState := DeviceData.State;
   			DeviceData.State := DeviceData.MaxState;
   			DeviceData.CommTimeOut := FALSE;
   			DeviceData.AcyclicData[0] := 0;
   			DeviceData.NewState := TRUE;
   
   		end_if;
   
   		//***************************************
   	    31: // Start zero point adjustment
   		//***************************************
   
   			CMD_Index := 2195;
   			CMD_Subindex := 0;
   			CMD_Wr := TRUE;	// Only Read or Write can be active
   			CMD_Rd := FALSE;
   			CMD_ByteLength := 2;	//Check Length
   			DataToSend[6] := 0;
   			DataToSend[7] := 0;
   			DataToSend[6].8 :=1;
   
   			Trigger := TRUE;
   
   			if DeviceData.NewState then
   
   				DeviceData.StateDone := TRUE;
   
   			end_if;
   
   			if  DeviceData.CommSuccess and DeviceData.ReplayIndex = CMD_Index then
   
   				Trigger := FALSE;
   				DeviceData.OldState := DeviceData.State;
   				DeviceData.State := DeviceData.State + 1;
   				DeviceData.CommSuccess := FALSE;
   				DeviceData.AcyclicData[0] := 0;
   				DeviceData.NewState := TRUE;
   
   			elsif DeviceData.CommTimeOut then
   
   				temp_string1 := 'Error in step ';
   				Temp_DINT := DeviceData.State;
   				DTOS(Temp_DINT, temp_string2);
   				CONCAT(temp_string1, temp_string2, qAOI_Diagnostic_String);
   
   				DeviceData.OldState := DeviceData.State;
   				DeviceData.State := DeviceData.MaxState;	//Check State
   				DeviceData.CommTimeOut := FALSE;
   				DeviceData.AcyclicData[0] := 0;
   				DeviceData.NewState := TRUE;
   
   			end_if;
   
   		//***************************************
   	    32: // Intermediate state
   		//***************************************
   			TONR (StandardTimer);
   			StandardTimer.PRE := 2000;
   			StandardTimer.TimerEnable := onlyonce;
   
   			CMD_Index := 297;
   			CMD_Subindex := 0;
   			CMD_Wr := FALSE;
   			CMD_Rd := TRUE;
   			CMD_ByteLength := 4;
   			DataToSend[6]:= 0;
   			DataToSend[7]:= 0;
   			Trigger := TRUE;
   
   			if DeviceData.NewState and not onlyonce then
   				DeviceData.StateDone := TRUE;
   			end_if;
   
   			if  DeviceData.CommSuccess and DeviceData.ReplayIndex = CMD_Index and not onlyonce then
   				Trigger := 0;
   				DeviceData.CommSuccess := FALSE;
   				DeviceData.AcyclicData[0] := 0;
   				DeviceData.NewState := TRUE;
   				onlyonce := TRUE;
   			end_if;
   
   			if StandardTimer.DN and onlyonce then
   				onlyonce := FALSE;
   				DeviceData.OldState := DeviceData.State;
   				DeviceData.State := DeviceData.State + 1;
   
   			end_if;
   
   		//***************************************
   	    33: // Read progress
   		//***************************************
   
   			CMD_Index := 2155;
   			CMD_Subindex := 0;
   			CMD_Wr := FALSE;
   			CMD_Rd := TRUE;
   			CMD_ByteLength := 2;
   			Trigger := TRUE;
   
   			if DeviceData.NewState then
   
   				DeviceData.StateDone := TRUE;
   
   			end_if;
   
   			if  DeviceData.CommSuccess and DeviceData.ReplayIndex = CMD_Index then
   
   				qReadProgress.0	:= DeviceData.AcyclicData[0].0;
   				qReadProgress.1	:= DeviceData.AcyclicData[0].1;
   				qReadProgress.2	:= DeviceData.AcyclicData[0].2;
   				qReadProgress.3	:= DeviceData.AcyclicData[0].3;
   				qReadProgress.4	:= DeviceData.AcyclicData[0].4;
   				qReadProgress.5	:= DeviceData.AcyclicData[0].5;
   				qReadProgress.6	:= DeviceData.AcyclicData[0].6;
   				qReadProgress.7	:= DeviceData.AcyclicData[0].7;
   
   				// Check if progress at 100 percent
   				if qReadProgress < 100 then
   
   					DeviceData.OldState := DeviceData.State - 2;
   					DeviceData.State := DeviceData.State - 1;
   					qZeroPointStatus := 8;
   
   				elsif qReadProgress = 100 then
   
   					DeviceData.OldState := DeviceData.State;
   					DeviceData.State := DeviceData.State + 1;
   
   				end_if;
   
   				Trigger := FALSE;
   				DeviceData.CommSuccess := FALSE;
   				DeviceData.AcyclicData[0] := 0;
   				DeviceData.NewState := TRUE;
   
   			elsif DeviceData.CommTimeOut then
   
   				temp_string1 := 'Error in step ';
   				Temp_DINT := DeviceData.State;
   				DTOS(Temp_DINT, temp_string2);
   				CONCAT(temp_string1, temp_string2, qAOI_Diagnostic_String);
   
   				DeviceData.OldState := DeviceData.State;
   				DeviceData.State := DeviceData.MaxState;
   				DeviceData.CommTimeOut := FALSE;
   				DeviceData.AcyclicData[0] := 0;
   				DeviceData.NewState := TRUE;
   
   			end_if;
   
   		//***************************************
   	    34: // Read zero point adjustment status
   		//***************************************
   
   			CMD_Index := 2196;
   			CMD_Subindex := 0;
   			CMD_Wr := 0;
   			CMD_Rd := TRUE;
   			CMD_ByteLength := 2;
   			Trigger := TRUE;
   
   			if DeviceData.NewState then
   
   				DeviceData.StateDone := TRUE;
   
   			end_if;
   
   			if  DeviceData.CommSuccess and DeviceData.ReplayIndex = CMD_Index then
   
   				qZeroPointStatus := DeviceData.AcyclicData[0];
   
   				if DeviceData.AcyclicData[0] = 8 then
   
   					qAOI_Diagnostic_String := 'Zero point adjustement already in progress';
   					DeviceData.OldState := DeviceData.State;
   					DeviceData.State := DeviceData.MaxState;
   
   				elsif DeviceData.AcyclicData[0] = 2 then
   
   					qAOI_Diagnostic_String := 'Zero point adjustement failed';
   					DeviceData.OldState := DeviceData.State;
   					DeviceData.State := DeviceData.MaxState;
   
   				elsif DeviceData.AcyclicData[0] = 5 then
   
   					qAOI_Diagnostic_String := 'Zero point adjustement done';
   					DeviceData.OldState := DeviceData.State;
   					DeviceData.State :=  DeviceData.MaxState;
   
   				end_if;
   
   				Trigger := FALSE;
   				DeviceData.CommSuccess := FALSE;
   				DeviceData.AcyclicData[0] := 0;
   				DeviceData.NewState := TRUE;
   
   			elsif DeviceData.CommTimeOut then
   
   				temp_string1 := 'Error in step ';
   				Temp_DINT := DeviceData.State;
   				DTOS(Temp_DINT, temp_string2);
   				CONCAT(temp_string1, temp_string2, qAOI_Diagnostic_String);
   
   				DeviceData.OldState := DeviceData.State;
   				DeviceData.State := DeviceData.MaxState;
   				DeviceData.CommTimeOut := FALSE;
   				DeviceData.AcyclicData[0] := 0;
   				DeviceData.NewState := TRUE;
   
   		end_if;
   
   		//*********************************
   		90: // Active diagnostic
   		//*********************************
   
   			CMD_Index := 297;
   			CMD_Subindex := 0;
   			CMD_Wr := FALSE;
   			CMD_Rd := TRUE;
   			CMD_ByteLength := 4;
   			Trigger := TRUE;
   
   			if DeviceData.NewState then
   				DeviceData.StateDone := TRUE;
   			end_if;
   
   			if  DeviceData.CommSuccess and DeviceData.ReplayIndex = CMD_Index then
   
   				qActual_Diagnostics_Code	:= DeviceData.AcyclicData[0];
   
   				case qActual_Diagnostics_Code of
   
   					0:
   						qActual_Diagnostics_String := '--------';
   					16777296:
   						qActual_Diagnostics_String := 'F910 Tubes not oscillating';
   					16777312:
   						qActual_Diagnostics_String := 'F437 Configuration incompatible';
   					16777319:
   						qActual_Diagnostics_String := 'F242 Firmware incompatible';
   					16777323:
   						qActual_Diagnostics_String := 'F252 Module incompatible';
   					16777337:
   						qActual_Diagnostics_String := 'F272 Electronic module faulty';
   					16777340:
   						qActual_Diagnostics_String := 'F270 Main electronics defective';
   					16777341:
   						qActual_Diagnostics_String := 'F271 Main electronics faulty';
   					16777354:
   						qActual_Diagnostics_String := 'F442 Frequency output saturated';
   					16777355:
   						qActual_Diagnostics_String := 'F410 Data transfer failed';
   					16777356:
   						qActual_Diagnostics_String := 'F443 Pulse output saturated';
   					16777361:
   						qActual_Diagnostics_String := 'F842 Process value below limit';
   					16777362:
   						qActual_Diagnostics_String := 'F862 Partly filled pipe';
   					16777375:
   						qActual_Diagnostics_String := 'F270 Main electronics defective';
   					16777376:
   						qActual_Diagnostics_String := 'F083 Memory content inconsistent';
   					16777412:
   						qActual_Diagnostics_String := 'F912 Medium inhomogeneous';
   					16777413:
   						qActual_Diagnostics_String := 'F834 Process temperature too high';
   					16777414:
   						qActual_Diagnostics_String := 'F835 Process temperature too low';
   					16777416:
   						qActual_Diagnostics_String := 'F046 Sensor limit exceeded';
   					16777418:
   						qActual_Diagnostics_String := 'F046 Sensor limit exceeded';
   					16777421:
   						qActual_Diagnostics_String := 'F913 Medium unsuitable';
   					16777422:
   						qActual_Diagnostics_String := 'F374 Electronic module faulty';
   					16777429:
   						qActual_Diagnostics_String := 'F022 Temperature sensor defective';
   					16777430:
   						qActual_Diagnostics_String := 'F022 Temperature sensor defective';
   					16777434:
   						qActual_Diagnostics_String := 'F372 Electronic module faulty';
   					16777435:
   						qActual_Diagnostics_String := 'F062 Sensor connection faulty';
   					16777436:
   						qActual_Diagnostics_String := 'F062 Sensor connection faulty';
   					16777439:
   						qActual_Diagnostics_String := 'F912 Medium inhomogeneous';
   					16777441:
   						qActual_Diagnostics_String := 'F283 Memory content inconsistent';
   					16777445:
   						qActual_Diagnostics_String := 'F273 Main electronics defective';
   					16777447:
   						qActual_Diagnostics_String := 'F082 Data storage inconsistent';
   					16777491:
   						qActual_Diagnostics_String := 'F062 Sensor connection faulty';
   					16777492:
   						qActual_Diagnostics_String := 'F062 Sensor connection faulty';
   					16777493:
   						qActual_Diagnostics_String := 'F912 Medium inhomogeneous';
   					16777504:
   						qActual_Diagnostics_String := 'F372 Electronic module faulty';
   					16777505:
   						qActual_Diagnostics_String := 'F443 Pulse output saturated';
   					16777506:
   						qActual_Diagnostics_String := 'F442 Frequency output saturated';
   					16777547:
   						qActual_Diagnostics_String := 'F201 Electronics faulty';
   					16777570:
   						qActual_Diagnostics_String := 'F912 Medium inhomogeneous';
   					16777576:
   						qActual_Diagnostics_String := 'F948 Oscillation damping too high';
   					16777583:
   						qActual_Diagnostics_String := 'F283 Memory content inconsistent';
   					16777930:
   						qActual_Diagnostics_String := 'F331 Firmware update failed in module 1';
   					16778273:
   						qActual_Diagnostics_String := 'F230 Date/time incorrect';
   					16778381:
   						qActual_Diagnostics_String := 'F231 Date/time not available';
   					16778382:
   						qActual_Diagnostics_String := 'F230 Date/time incorrect';
   					16778490:
   						qActual_Diagnostics_String := 'F419 Power cycle required';
   					16843466:
   						qActual_Diagnostics_String := 'F331 Firmware update failed in module 2';
   					33554570:
   						qActual_Diagnostics_String := 'C442 Frequency output saturated';
   					33554572:
   						qActual_Diagnostics_String := 'C443 Pulse output saturated';
   					33554573:
   						qActual_Diagnostics_String := 'C492 Frequency output simulation active';
   					33554574:
   						qActual_Diagnostics_String := 'C493 Pulse output simulation active';
   					33554575:
   						qActual_Diagnostics_String := 'C494 Switch output simulation active';
   					33554576:
   						qActual_Diagnostics_String := 'C484 Failure mode simulation active';
   					33554577:
   						qActual_Diagnostics_String := 'C842 Process value below limit';
   					33554578:
   						qActual_Diagnostics_String := 'C862 Partly filled pipe';
   					33554579:
   						qActual_Diagnostics_String := 'C485 Process variable simulation active';
   					33554580:
   						qActual_Diagnostics_String := 'C453 Flow override active';
   					33554628:
   						qActual_Diagnostics_String := 'C912 Medium inhomogeneous';
   					33554629:
   						qActual_Diagnostics_String := 'C834 Process temperature too high';
   					33554630:
   						qActual_Diagnostics_String := 'C835 Process temperature too low';
   					33554632:
   						qActual_Diagnostics_String := 'C046 Sensor limit exceeded';
   					33554634:
   						qActual_Diagnostics_String := 'C046 Sensor limit exceeded';
   					33554637:
   						qActual_Diagnostics_String := 'C913 Medium unsuitable';
   					33554638:
   						qActual_Diagnostics_String := 'C374 Electronic module faulty';
   					33554655:
   						qActual_Diagnostics_String := 'C912 Medium inhomogeneous';
   					33554709:
   						qActual_Diagnostics_String := 'C912 Medium inhomogeneous';
   					33554721:
   						qActual_Diagnostics_String := 'C443 Pulse output saturated';
   					33554722:
   						qActual_Diagnostics_String := 'C442 Frequency output saturated';
   					33554782:
   						qActual_Diagnostics_String := 'C495 Diagnostic event simulation active';
   					33554786:
   						qActual_Diagnostics_String := 'C912 Medium inhomogeneous';
   					33554792:
   						qActual_Diagnostics_String := 'C948 Oscillation damping too high';
   					33554948:
   						qActual_Diagnostics_String := 'C412 Processing download';
   					33555489:
   						qActual_Diagnostics_String := 'C230 Date/time incorrect';
   					33555597:
   						qActual_Diagnostics_String := 'C231 Date/time not available';
   					33555598:
   						qActual_Diagnostics_String := 'C230 Date/time incorrect';
   					67108970:
   						qActual_Diagnostics_String := 'M438 Dataset different';
   					67109002:
   						qActual_Diagnostics_String := 'M442 Frequency output saturated';
   					67109004:
   						qActual_Diagnostics_String := 'M443 Pulse output saturated';
   					67109009:
   						qActual_Diagnostics_String := 'M842 Process value below limit';
   					67109010:
   						qActual_Diagnostics_String := 'M862 Partly filled pipe';
   					67109060:
   						qActual_Diagnostics_String := 'M912 Medium inhomogeneous';
   					67109061:
   						qActual_Diagnostics_String := 'M834 Process temperature too high';
   					67109062:
   						qActual_Diagnostics_String := 'M835 Process temperature too low';
   					67109064:
   						qActual_Diagnostics_String := 'M046 Sensor limit exceeded';
   					67109066:
   						qActual_Diagnostics_String := 'M046 Sensor limit exceeded';
   					67109069:
   						qActual_Diagnostics_String := 'M913 Medium unsuitable';
   					67109070:
   						qActual_Diagnostics_String := 'M374 Electronic module faulty';
   					67109087:
   						qActual_Diagnostics_String := 'M912 Medium inhomogeneous';
   					67109090:
   						qActual_Diagnostics_String := 'M311 Electronic module faulty';
   					67109141:
   						qActual_Diagnostics_String := 'M912 Medium inhomogeneous';
   					67109153:
   						qActual_Diagnostics_String := 'M443 Pulse output saturated';
   					67109154:
   						qActual_Diagnostics_String := 'M442 Frequency output saturated';
   					67109218:
   						qActual_Diagnostics_String := 'M912 Medium inhomogeneous';
   					67109224:
   						qActual_Diagnostics_String := 'M948 Oscillation damping too high';
   					67109921:
   						qActual_Diagnostics_String := 'M230 Date/time incorrect';
   					67110029:
   						qActual_Diagnostics_String := 'M231 Date/time not available';
   					67110030:
   						qActual_Diagnostics_String := 'M230 Date/time incorrect';
   					134217866:
   						qActual_Diagnostics_String := 'S442 Frequency output saturated';
   					134217868:
   						qActual_Diagnostics_String := 'S443 Pulse output saturated';
   					134217873:
   						qActual_Diagnostics_String := 'S842 Process value below limit';
   					134217874:
   						qActual_Diagnostics_String := 'S862 Partly filled pipe';
   					134217924:
   						qActual_Diagnostics_String := 'S912 Medium inhomogeneous';
   					134217925:
   						qActual_Diagnostics_String := 'S834 Process temperature too high';
   					134217926:
   						qActual_Diagnostics_String := 'S835 Process temperature too low';
   					134217928:
   						qActual_Diagnostics_String := 'S046 Sensor limit exceeded';
   					134217930:
   						qActual_Diagnostics_String := 'S046 Sensor limit exceeded';
   					134217932:
   						qActual_Diagnostics_String := 'S140 Sensor signal asymmetrical';
   					134217933:
   						qActual_Diagnostics_String := 'S913 Medium unsuitable';
   					134217934:
   						qActual_Diagnostics_String := 'S374 Electronic module faulty';
   					134217951:
   						qActual_Diagnostics_String := 'S912 Medium inhomogeneous';
   					134218005:
   						qActual_Diagnostics_String := 'S912 Medium inhomogeneous';
   					134218017:
   						qActual_Diagnostics_String := 'S443 Pulse output saturated';
   					134218018:
   						qActual_Diagnostics_String := 'S442 Frequency output saturated';
   					134218082:
   						qActual_Diagnostics_String := 'S912 Medium inhomogeneous';
   					134218088:
   						qActual_Diagnostics_String := 'S948 Oscillation damping too high';
   					134218785:
   						qActual_Diagnostics_String := 'S230 Date/time incorrect';
   					134218893:
   						qActual_Diagnostics_String := 'S231 Date/time not available';
   					134218894:
   						qActual_Diagnostics_String := 'S230 Date/time incorrect';
   					134219072:
   						qActual_Diagnostics_String := 'S880 Output overloaded';
   					536871050:
   						qActual_Diagnostics_String := '442 Frequency output saturated';
   					536871052:
   						qActual_Diagnostics_String := '443 Pulse output saturated';
   					536871057:
   						qActual_Diagnostics_String := '842 Process value below limit';
   					536871058:
   						qActual_Diagnostics_String := '862 Partly filled pipe';
   					536871108:
   						qActual_Diagnostics_String := '912 Medium inhomogeneous';
   					536871109:
   						qActual_Diagnostics_String := '834 Process temperature too high';
   					536871110:
   						qActual_Diagnostics_String := '835 Process temperature too low';
   					536871112:
   						qActual_Diagnostics_String := '046 Sensor limit exceeded';
   					536871114:
   						qActual_Diagnostics_String := '046 Sensor limit exceeded';
   					536871117:
   						qActual_Diagnostics_String := '913 Medium unsuitable';
   					536871118:
   						qActual_Diagnostics_String := '374 Electronic module faulty';
   					536871135:
   						qActual_Diagnostics_String := '912 Medium inhomogeneous';
   					536871189:
   						qActual_Diagnostics_String := '912 Medium inhomogeneous';
   					536871201:
   						qActual_Diagnostics_String := '443 Pulse output saturated';
   					536871202:
   						qActual_Diagnostics_String := '442 Frequency output saturated';
   					536871266:
   						qActual_Diagnostics_String := '912 Medium inhomogeneous';
   					536871272:
   						qActual_Diagnostics_String := '948 Oscillation damping too high';
   					536871969:
   						qActual_Diagnostics_String := '230 Date/time incorrect';
   					536872077:
   						qActual_Diagnostics_String := '231 Date/time not available';
   					536872078:
   						qActual_Diagnostics_String := '230 Date/time incorrect';
   				else
   
   					qActual_Diagnostics_String := 'Error Code unknown';
   
   				end_case;
   
   				Trigger := FALSE;
   				DeviceData.OldState := DeviceData.State;
   		        DeviceData.State := DeviceData.State + 1;
   				DeviceData.CommSuccess := FALSE;
   				DeviceData.AcyclicData[0] := 0;
   				DeviceData.NewState := TRUE;
   
   
   
   			 elsif DeviceData.CommTimeOut then
   
   				temp_string1 := 'Error in step ';
   				Temp_DINT := DeviceData.State;
   				DTOS(Temp_DINT, temp_string2);
   				CONCAT(temp_string1, temp_string2, qAOI_Diagnostic_String);
   
   				DeviceData.OldState := DeviceData.State;
   				DeviceData.State := DeviceData.MaxState;	//Check State
   				DeviceData.CommTimeOut := FALSE;
   				DeviceData.AcyclicData[0] := 0;
   				DeviceData.NewState := TRUE;
   
   		    end_if;
   
   		//*********************************
   	    91: // Previous Diagnostic
   	    //*********************************
   
   		    CMD_Index := 298;
   			CMD_Subindex := 0;
   		    CMD_Wr := FALSE;
   			CMD_Rd := TRUE;
   			CMD_ByteLength := 4;
   			Trigger := TRUE;
   
   			if DeviceData.NewState then
   				DeviceData.StateDone := TRUE;
   			end_if;
   
   			if  DeviceData.CommSuccess and DeviceData.ReplayIndex = CMD_Index then
   
   				qLast_Diagnostics_Code	:= DeviceData.AcyclicData[0];
   
   				case qLast_Diagnostics_Code of
   
   										0:
   						qLast_Diagnostics_String := '--------';
   					16777296:
   						qLast_Diagnostics_String := 'F910 Tubes not oscillating';
   					16777312:
   						qLast_Diagnostics_String := 'F437 Configuration incompatible';
   					16777319:
   						qLast_Diagnostics_String := 'F242 Firmware incompatible';
   					16777323:
   						qLast_Diagnostics_String := 'F252 Module incompatible';
   					16777337:
   						qLast_Diagnostics_String := 'F272 Electronic module faulty';
   					16777340:
   						qLast_Diagnostics_String := 'F270 Main electronics defective';
   					16777341:
   						qLast_Diagnostics_String := 'F271 Main electronics faulty';
   					16777354:
   						qLast_Diagnostics_String := 'F442 Frequency output saturated';
   					16777355:
   						qLast_Diagnostics_String := 'F410 Data transfer failed';
   					16777356:
   						qLast_Diagnostics_String := 'F443 Pulse output saturated';
   					16777361:
   						qLast_Diagnostics_String := 'F842 Process value below limit';
   					16777362:
   						qLast_Diagnostics_String := 'F862 Partly filled pipe';
   					16777375:
   						qLast_Diagnostics_String := 'F270 Main electronics defective';
   					16777376:
   						qLast_Diagnostics_String := 'F083 Memory content inconsistent';
   					16777412:
   						qLast_Diagnostics_String := 'F912 Medium inhomogeneous';
   					16777413:
   						qLast_Diagnostics_String := 'F834 Process temperature too high';
   					16777414:
   						qLast_Diagnostics_String := 'F835 Process temperature too low';
   					16777416:
   						qLast_Diagnostics_String := 'F046 Sensor limit exceeded';
   					16777418:
   						qLast_Diagnostics_String := 'F046 Sensor limit exceeded';
   					16777421:
   						qLast_Diagnostics_String := 'F913 Medium unsuitable';
   					16777422:
   						qLast_Diagnostics_String := 'F374 Electronic module faulty';
   					16777429:
   						qLast_Diagnostics_String := 'F022 Temperature sensor defective';
   					16777430:
   						qLast_Diagnostics_String := 'F022 Temperature sensor defective';
   					16777434:
   						qLast_Diagnostics_String := 'F372 Electronic module faulty';
   					16777435:
   						qLast_Diagnostics_String := 'F062 Sensor connection faulty';
   					16777436:
   						qLast_Diagnostics_String := 'F062 Sensor connection faulty';
   					16777439:
   						qLast_Diagnostics_String := 'F912 Medium inhomogeneous';
   					16777441:
   						qLast_Diagnostics_String := 'F283 Memory content inconsistent';
   					16777445:
   						qLast_Diagnostics_String := 'F273 Main electronics defective';
   					16777447:
   						qLast_Diagnostics_String := 'F082 Data storage inconsistent';
   					16777491:
   						qLast_Diagnostics_String := 'F062 Sensor connection faulty';
   					16777492:
   						qLast_Diagnostics_String := 'F062 Sensor connection faulty';
   					16777493:
   						qLast_Diagnostics_String := 'F912 Medium inhomogeneous';
   					16777504:
   						qLast_Diagnostics_String := 'F372 Electronic module faulty';
   					16777505:
   						qLast_Diagnostics_String := 'F443 Pulse output saturated';
   					16777506:
   						qLast_Diagnostics_String := 'F442 Frequency output saturated';
   					16777547:
   						qLast_Diagnostics_String := 'F201 Electronics faulty';
   					16777570:
   						qLast_Diagnostics_String := 'F912 Medium inhomogeneous';
   					16777576:
   						qLast_Diagnostics_String := 'F948 Oscillation damping too high';
   					16777583:
   						qLast_Diagnostics_String := 'F283 Memory content inconsistent';
   					16777930:
   						qLast_Diagnostics_String := 'F331 Firmware update failed in module 1';
   					16778273:
   						qLast_Diagnostics_String := 'F230 Date/time incorrect';
   					16778381:
   						qLast_Diagnostics_String := 'F231 Date/time not available';
   					16778382:
   						qLast_Diagnostics_String := 'F230 Date/time incorrect';
   					16778490:
   						qLast_Diagnostics_String := 'F419 Power cycle required';
   					16843466:
   						qLast_Diagnostics_String := 'F331 Firmware update failed in module 2';
   					33554570:
   						qLast_Diagnostics_String := 'C442 Frequency output saturated';
   					33554572:
   						qLast_Diagnostics_String := 'C443 Pulse output saturated';
   					33554573:
   						qLast_Diagnostics_String := 'C492 Frequency output simulation active';
   					33554574:
   						qLast_Diagnostics_String := 'C493 Pulse output simulation active';
   					33554575:
   						qLast_Diagnostics_String := 'C494 Switch output simulation active';
   					33554576:
   						qLast_Diagnostics_String := 'C484 Failure mode simulation active';
   					33554577:
   						qLast_Diagnostics_String := 'C842 Process value below limit';
   					33554578:
   						qLast_Diagnostics_String := 'C862 Partly filled pipe';
   					33554579:
   						qLast_Diagnostics_String := 'C485 Process variable simulation active';
   					33554580:
   						qLast_Diagnostics_String := 'C453 Flow override active';
   					33554628:
   						qLast_Diagnostics_String := 'C912 Medium inhomogeneous';
   					33554629:
   						qLast_Diagnostics_String := 'C834 Process temperature too high';
   					33554630:
   						qLast_Diagnostics_String := 'C835 Process temperature too low';
   					33554632:
   						qLast_Diagnostics_String := 'C046 Sensor limit exceeded';
   					33554634:
   						qLast_Diagnostics_String := 'C046 Sensor limit exceeded';
   					33554637:
   						qLast_Diagnostics_String := 'C913 Medium unsuitable';
   					33554638:
   						qLast_Diagnostics_String := 'C374 Electronic module faulty';
   					33554655:
   						qLast_Diagnostics_String := 'C912 Medium inhomogeneous';
   					33554709:
   						qLast_Diagnostics_String := 'C912 Medium inhomogeneous';
   					33554721:
   						qLast_Diagnostics_String := 'C443 Pulse output saturated';
   					33554722:
   						qLast_Diagnostics_String := 'C442 Frequency output saturated';
   					33554782:
   						qLast_Diagnostics_String := 'C495 Diagnostic event simulation active';
   					33554786:
   						qLast_Diagnostics_String := 'C912 Medium inhomogeneous';
   					33554792:
   						qLast_Diagnostics_String := 'C948 Oscillation damping too high';
   					33554948:
   						qLast_Diagnostics_String := 'C412 Processing download';
   					33555489:
   						qLast_Diagnostics_String := 'C230 Date/time incorrect';
   					33555597:
   						qLast_Diagnostics_String := 'C231 Date/time not available';
   					33555598:
   						qLast_Diagnostics_String := 'C230 Date/time incorrect';
   					67108970:
   						qLast_Diagnostics_String := 'M438 Dataset different';
   					67109002:
   						qLast_Diagnostics_String := 'M442 Frequency output saturated';
   					67109004:
   						qLast_Diagnostics_String := 'M443 Pulse output saturated';
   					67109009:
   						qLast_Diagnostics_String := 'M842 Process value below limit';
   					67109010:
   						qLast_Diagnostics_String := 'M862 Partly filled pipe';
   					67109060:
   						qLast_Diagnostics_String := 'M912 Medium inhomogeneous';
   					67109061:
   						qLast_Diagnostics_String := 'M834 Process temperature too high';
   					67109062:
   						qLast_Diagnostics_String := 'M835 Process temperature too low';
   					67109064:
   						qLast_Diagnostics_String := 'M046 Sensor limit exceeded';
   					67109066:
   						qLast_Diagnostics_String := 'M046 Sensor limit exceeded';
   					67109069:
   						qLast_Diagnostics_String := 'M913 Medium unsuitable';
   					67109070:
   						qLast_Diagnostics_String := 'M374 Electronic module faulty';
   					67109087:
   						qLast_Diagnostics_String := 'M912 Medium inhomogeneous';
   					67109090:
   						qLast_Diagnostics_String := 'M311 Electronic module faulty';
   					67109141:
   						qLast_Diagnostics_String := 'M912 Medium inhomogeneous';
   					67109153:
   						qLast_Diagnostics_String := 'M443 Pulse output saturated';
   					67109154:
   						qLast_Diagnostics_String := 'M442 Frequency output saturated';
   					67109218:
   						qLast_Diagnostics_String := 'M912 Medium inhomogeneous';
   					67109224:
   						qLast_Diagnostics_String := 'M948 Oscillation damping too high';
   					67109921:
   						qLast_Diagnostics_String := 'M230 Date/time incorrect';
   					67110029:
   						qLast_Diagnostics_String := 'M231 Date/time not available';
   					67110030:
   						qLast_Diagnostics_String := 'M230 Date/time incorrect';
   					134217866:
   						qLast_Diagnostics_String := 'S442 Frequency output saturated';
   					134217868:
   						qLast_Diagnostics_String := 'S443 Pulse output saturated';
   					134217873:
   						qLast_Diagnostics_String := 'S842 Process value below limit';
   					134217874:
   						qLast_Diagnostics_String := 'S862 Partly filled pipe';
   					134217924:
   						qLast_Diagnostics_String := 'S912 Medium inhomogeneous';
   					134217925:
   						qLast_Diagnostics_String := 'S834 Process temperature too high';
   					134217926:
   						qLast_Diagnostics_String := 'S835 Process temperature too low';
   					134217928:
   						qLast_Diagnostics_String := 'S046 Sensor limit exceeded';
   					134217930:
   						qLast_Diagnostics_String := 'S046 Sensor limit exceeded';
   					134217932:
   						qLast_Diagnostics_String := 'S140 Sensor signal asymmetrical';
   					134217933:
   						qLast_Diagnostics_String := 'S913 Medium unsuitable';
   					134217934:
   						qLast_Diagnostics_String := 'S374 Electronic module faulty';
   					134217951:
   						qLast_Diagnostics_String := 'S912 Medium inhomogeneous';
   					134218005:
   						qLast_Diagnostics_String := 'S912 Medium inhomogeneous';
   					134218017:
   						qLast_Diagnostics_String := 'S443 Pulse output saturated';
   					134218018:
   						qLast_Diagnostics_String := 'S442 Frequency output saturated';
   					134218082:
   						qLast_Diagnostics_String := 'S912 Medium inhomogeneous';
   					134218088:
   						qLast_Diagnostics_String := 'S948 Oscillation damping too high';
   					134218785:
   						qLast_Diagnostics_String := 'S230 Date/time incorrect';
   					134218893:
   						qLast_Diagnostics_String := 'S231 Date/time not available';
   					134218894:
   						qLast_Diagnostics_String := 'S230 Date/time incorrect';
   					134219072:
   						qLast_Diagnostics_String := 'S880 Output overloaded';
   					536871050:
   						qLast_Diagnostics_String := '442 Frequency output saturated';
   					536871052:
   						qLast_Diagnostics_String := '443 Pulse output saturated';
   					536871057:
   						qLast_Diagnostics_String := '842 Process value below limit';
   					536871058:
   						qLast_Diagnostics_String := '862 Partly filled pipe';
   					536871108:
   						qLast_Diagnostics_String := '912 Medium inhomogeneous';
   					536871109:
   						qLast_Diagnostics_String := '834 Process temperature too high';
   					536871110:
   						qLast_Diagnostics_String := '835 Process temperature too low';
   					536871112:
   						qLast_Diagnostics_String := '046 Sensor limit exceeded';
   					536871114:
   						qLast_Diagnostics_String := '046 Sensor limit exceeded';
   					536871117:
   						qLast_Diagnostics_String := '913 Medium unsuitable';
   					536871118:
   						qLast_Diagnostics_String := '374 Electronic module faulty';
   					536871135:
   						qLast_Diagnostics_String := '912 Medium inhomogeneous';
   					536871189:
   						qLast_Diagnostics_String := '912 Medium inhomogeneous';
   					536871201:
   						qLast_Diagnostics_String := '443 Pulse output saturated';
   					536871202:
   						qLast_Diagnostics_String := '442 Frequency output saturated';
   					536871266:
   						qLast_Diagnostics_String := '912 Medium inhomogeneous';
   					536871272:
   						qLast_Diagnostics_String := '948 Oscillation damping too high';
   					536871969:
   						qLast_Diagnostics_String := '230 Date/time incorrect';
   					536872077:
   						qLast_Diagnostics_String := '231 Date/time not available';
   					536872078:
   						qLast_Diagnostics_String := '230 Date/time incorrect';
   				else
   						qLast_Diagnostics_String := 'Error Code unknown';
   
   				end_case;
   
   				Trigger := FALSE;
   				DeviceData.OldState := DeviceData.State;
   		        DeviceData.State := DeviceData.MaxState;
   				DeviceData.CommSuccess := FALSE;
   				DeviceData.AcyclicData[0] := 0;
   				DeviceData.NewState := TRUE;
   
   			 elsif DeviceData.CommTimeOut then
   
   				temp_string1 := 'Error in step ';
   				Temp_DINT := DeviceData.State;
   				DTOS(Temp_DINT, temp_string2);
   				CONCAT(temp_string1, temp_string2, qAOI_Diagnostic_String);
   
   				DeviceData.OldState := DeviceData.State;
   				DeviceData.State := DeviceData.MaxState;	//Check State
   				DeviceData.CommTimeOut := FALSE;
   				DeviceData.AcyclicData[0] := 0;
   				DeviceData.NewState := TRUE;
   
   			end_if;
   
   		//*********************************
   		98: // End Step Trigger Guard
   		//*********************************
   
   				DeviceData.State := 0;
   				CommAOIBusy := 0;
   				DeviceAOISendRequest.[DeviceData.DevicePort] := FALSE;
   				ActiveComPort := 0;
   				ActiveAOI := FALSE;
   				DataToSend[0] := 0;
   				DataToSend[1] := 0;
   				DataToSend[2] := 0;
   				DataToSend[3] := 0;
   				DataToSend[4] := 0;
   				DataToSend[5] := 0;
    				DataToSend[6] := 0;
   				DataToSend[7] := 0;
    				DataToSend[8] := 0;
   				DataToSend[9] := 0;
   				DeviceData.StateDone := FALSE;
   				Skip := FALSE;
   				DeviceData.State := 0;
   				firstTimeDone := FALSE;
   				DeviceData.NewState := FALSE;
   				DeviceData.OldState := 0;
   				ActiveAOI := FALSE;
   
   				if PulseSimActive then
   
   					PulseSimActive := FALSE;
   					PulseSimChanged := FALSE;
   
   				elsif TotActive then
   
   					TotActive := FALSE;
   					TotChanged := FALSE;
   
   				elsif ZeroPointActive then
   
   					ZeroPointActive := FALSE;
   					StartZeroPointAdjustmentChanged := FALSE;
   
   				elsif ParameterizeActive then
   
   					ParameterizeActive := FALSE;
   					ParameterizeChanged := FALSE;
   
   				elsif CondStatusActive then
   
   					CondStatusActive := FALSE;
   					CondStatusChanged := FALSE;
   
   				end_if;
   
   	end_case;
   
   	end_if;
   
   	//*************************
   	// Execution Area
   	//*************************
   	if DeviceData.State > StateMin and DeviceData.State < DeviceData.MaxState then
   
   		DataToSend[2] := DeviceData.DevicePort;
   		DataToSend[3] := CMD_Index;
   		DataToSend[4] := CMD_Subindex;
   		DataToSend[5].0 := CMD_Rd;
   		DataToSend[5].1 := CMD_Wr;
   		DataToSend[5].8 := CMD_ByteLength.0;  // Bits for the Length of the Data
   		DataToSend[5].9 := CMD_ByteLength.1;
   		DataToSend[5].10 := CMD_ByteLength.2;
   		DataToSend[5].11 := CMD_ByteLength.3;
   		DataToSend[5].12 := CMD_ByteLength.4;
   		DataToSend[5].13 := CMD_ByteLength.5;
   		DataToSend[5].14 := CMD_ByteLength.6;
   		DataToSend[5].15 := CMD_ByteLength.7;
   		DataToSend[5].7 := Trigger;
   
   		qCommError := CommError;
   
   	end_if;
   
   
   end_if;
END_ROUTINE
END_ADD_ON_INSTRUCTION
